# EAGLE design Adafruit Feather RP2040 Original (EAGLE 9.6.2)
COMPANY: ADAFRUIT INDUSTRIES; DRAWN: KTOWN; REV: B
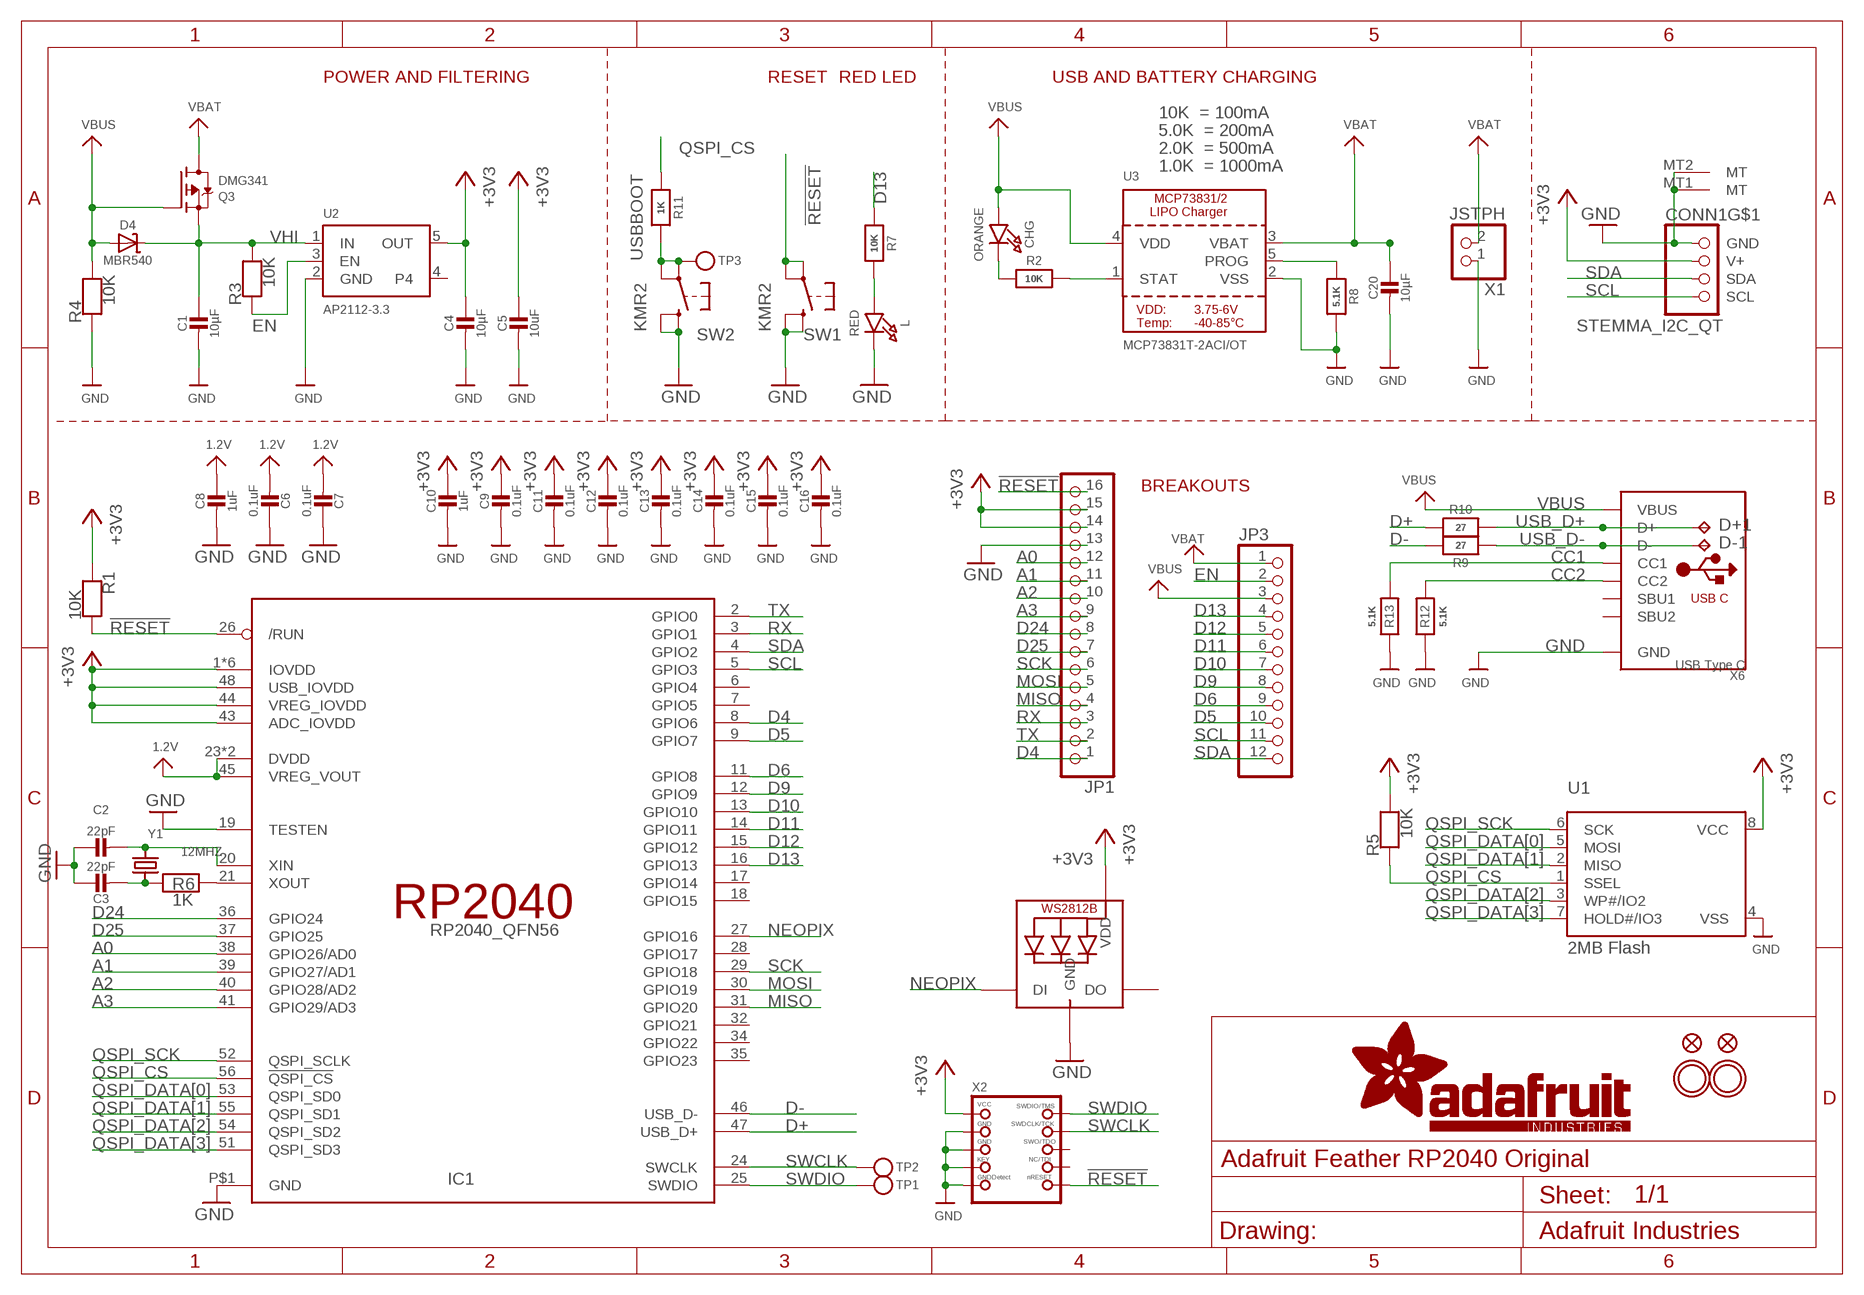
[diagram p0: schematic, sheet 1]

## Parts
C1  10µF  CAP_CERAMIC0805-NOOUTLINE  [0805-NO]
C2  22pF  CAP_CERAMIC0603_NO  [0603-NO]
C3  22pF  CAP_CERAMIC0603_NO  [0603-NO]
C4  10µF  CAP_CERAMIC0805-NOOUTLINE  [0805-NO]
C5  10uF  CAP_CERAMIC0805-NOOUTLINE  [0805-NO]
C6  0.1uF  CAP_CERAMIC0603_NO  [0603-NO]
C7  0.1uF  CAP_CERAMIC0603_NO  [0603-NO]
C8  1uF  CAP_CERAMIC0603_NO  [0603-NO]
C9  0.1uF  CAP_CERAMIC0603_NO  [0603-NO]
C10  1uF  CAP_CERAMIC0603_NO  [0603-NO]
C11  0.1uF  CAP_CERAMIC0603_NO  [0603-NO]
C12  0.1uF  CAP_CERAMIC0603_NO  [0603-NO]
C13  0.1uF  CAP_CERAMIC0603_NO  [0603-NO]
C14  0.1uF  CAP_CERAMIC0603_NO  [0603-NO]
C15  0.1uF  CAP_CERAMIC0603_NO  [0603-NO]
C16  0.1uF  CAP_CERAMIC0603_NO  [0603-NO]
C20  10µF  CAP_CERAMIC0805-NOOUTLINE  [0805-NO]
CHG  ORANGE  LED0603_NOOUTLINE  [CHIPLED_0603_NOOUTLINE]
CONN1  STEMMA_I2C_QT  [JST_SH4]
D4  MBR540  DIODE-SCHOTTKYSOD-123  [SOD-123]
D+1  TPB1,27  [B1,27]
D-1  TPB1,27  [B1,27]
IC1  RP2040_QFN56  [QFN56_7MM_REDUCEDEPAD]
JP1  HEADER-1X16ROUND  [1X16_ROUND]
JP3  HEADER-1X12  [1X12_ROUND]
L  RED  LED0603_NOOUTLINE  [CHIPLED_0603_NOOUTLINE]
LED1  WS2812B3535  [LED3535]
Q3  DMG341  MOSFET-P  [SOT23-R]
R1  10K  RESISTOR_0603_NOOUT  [0603-NO]
R2  10K  RESISTOR_0603_NOOUT  [0603-NO]
R3  10K  RESISTOR_0603_NOOUT  [0603-NO]
R4  10K  RESISTOR_0603_NOOUT  [0603-NO]
R5  10K  RESISTOR_0603_NOOUT  [0603-NO]
R6  1K  RESISTOR_0603_NOOUT  [0603-NO]
R7  10K  RESISTOR_0603_NOOUT  [0603-NO]
R8  5.1K  RESISTOR_0603_NOOUT  [0603-NO]
R9  27  RESISTOR_0603_NOOUT  [0603-NO]
R10  27  RESISTOR_0603_NOOUT  [0603-NO]
R11  1K  RESISTOR_0603_NOOUT  [0603-NO]
R12  5.1K  RESISTOR_0603_NOOUT  [0603-NO]
R13  5.1K  RESISTOR_0603_NOOUT  [0603-NO]
SW1  KMR2  SWITCH_TACT_SMT4.6X2.8  [BTN_KMR2_4.6X2.8]
SW2  KMR2  SWITCH_TACT_SMT4.6X2.8  [BTN_KMR2_4.6X2.8]
TP1  TESTPOINTROUND1.5MMNO  [TESTPOINT_ROUND_1.5MM_NO]
TP2  TESTPOINTROUND1.5MMNO  [TESTPOINT_ROUND_1.5MM_NO]
TP3  TESTPOINTROUND1.5MMNO  [TESTPOINT_ROUND_1.5MM_NO]
U1  2MB Flash  SPIFLASH_8PIN208MIL  [SOIC8_208MIL]
U2  AP2112-3.3  VREG_SOT23-5  [SOT23-5@1]
U3  MCP73831T-2ACI/OT  MCP73831/2  [SOT23-5]
U$31  MOUNTINGHOLE2.5  [MOUNTINGHOLE_2.5_PLATED]
U$32  MOUNTINGHOLE2.5  [MOUNTINGHOLE_2.5_PLATED]
U$34  FIDUCIAL_1MM  [FIDUCIAL_1MM]
U$35  FIDUCIAL_1MM  [FIDUCIAL_1MM]
X1  JSTPH  CON_JST_PH_2PIN_BATT  [JSTPH2_BATT]
X2  JTAG-CORTEXBOXPOSTS  [2X05_1.27MM_BOX_POSTS]
X6  USB Type C  USB_C  [USB_C_CUSB31-CFM2AX-01-X]
Y1  12MHZ  CRYSTAL2.5X2.0  [CRYSTAL_2.5X2]

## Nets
1.2V: C6.2 C7.2 C8.1 IC1.23(DVDD) IC1.45(VREG_VOUT) IC1.50(DVDD)
!RESET: IC1.26(/RUN) JP1.16 R1.2 SW1.A'(P1) SW1.A(P) X2.10(NRESET)
+3V3: C4.1 C5.1 C9.1 C10.1 C11.1 C12.1 C13.1 C14.1 C15.1 C16.1 CONN1.2(V+) IC1.1(IOVDD) IC1.10(IOVDD) IC1.22(IOVDD) IC1.33(IOVDD) IC1.42(IOVDD) IC1.43(ADC_IOVDD) IC1.44(VREG_IOVDD) IC1.48(USB_IOVDD) IC1.49(IOVDD) JP1.14 JP1.15 LED1.2(VDD) R1.1 R5.2 U1.8(VCC) U2.5(OUT) X2.1(VCC)
A0: IC1.38(GPIO26/AD0) JP1.12
A1: IC1.39(GPIO27/AD1) JP1.11
A2: IC1.40(GPIO28/AD2) JP1.10
A3: IC1.41(GPIO29/AD3) JP1.9
CC1: R13.2 X6.A5(CC1)
CC2: R12.2 X6.B5(CC2)
D4: IC1.8(GPIO6) JP1.1
D5: IC1.9(GPIO7) JP3.10
D6: IC1.11(GPIO8) JP3.9
D9: IC1.12(GPIO9) JP3.8
D10: IC1.13(GPIO10) JP3.7
D11: IC1.14(GPIO11) JP3.6
D12: IC1.15(GPIO12) JP3.5
D13: IC1.16(GPIO13) JP3.4 R7.1
D24: IC1.36(GPIO24) JP1.8
D25: IC1.37(GPIO25) JP1.7
D+: IC1.47(USB_D+) R10.2
D-: IC1.46(USB_D-) R9.2
EN: JP3.2 R3.1 U2.3(EN)
GND [power]: C1.2 C2.1 C3.1 C4.2 C5.2 C6.1 C7.1 C8.2 C9.2 C10.2 C11.2 C12.2 C13.2 C14.2 C15.2 C16.2 C20.2 CONN1.1(GND) CONN1.MT1(MT) CONN1.MT2(MT) IC1.19(TESTEN) IC1.P$1(GND) JP1.13 L.C LED1.4(GND) R4.1 R8.2 R12.1 R13.1 SW1.B'(S1) SW1.B(S) SW2.B'(S1) SW2.B(S) U1.4(VSS) U2.2(GND) U3.2(VSS) X1.1 X2.3(GND) X2.5(GND) X2.7(KEY) X2.9(GNDDETECT) X6.A1B12(GND) X6.B1A12(GND)
MISO: IC1.31(GPIO20) JP1.4
MOSI: IC1.30(GPIO19) JP1.5
N$1: CHG.C R2.1
N$2: L.A R7.2
N$3: R2.2 U3.1(STAT)
N$4: R8.1 U3.5(PROG)
N$5: C2.2 IC1.20(XIN) Y1.3
N$6: C3.2 R6.1 Y1.1
N$7: IC1.21(XOUT) R6.2
NEOPIX: IC1.27(GPIO16) LED1.1(DI)
QSPI_CS: IC1.56(!QSPI_CS) R5.1 R11.1 U1.1(SSEL)
QSPI_DATA[0]: IC1.53(QSPI_SD0) U1.5(MOSI)
QSPI_DATA[1]: IC1.55(QSPI_SD1) U1.2(MISO)
QSPI_DATA[2]: IC1.54(QSPI_SD2) U1.3(WP#/IO2)
QSPI_DATA[3]: IC1.51(QSPI_SD3) U1.7(HOLD#/IO3)
QSPI_SCK: IC1.52(QSPI_SCLK) U1.6(SCK)
RX: IC1.3(GPIO1) JP1.3
SCK: IC1.29(GPIO18) JP1.6
SCL: CONN1.4(SCL) IC1.5(GPIO3) JP3.11
SDA: CONN1.3(SDA) IC1.4(GPIO2) JP3.12
SWCLK: IC1.24(SWCLK) TP2.P$1 X2.4(SWDCLK)
SWDIO: IC1.25(SWDIO) TP1.P$1 X2.2(SWDIO)
TX: IC1.2(GPIO0) JP1.2
USB_D+: D+1.TP R10.1 X6.A6(D+) X6.B6(D+)
USB_D-: D-1.TP R9.1 X6.A7(D-) X6.B7(D-)
USBBOOT: R11.2 SW2.A'(P1) SW2.A(P) TP3.P$1
VBAT [power]: C20.1 JP3.1 Q3.3(D) U3.3(VBAT) X1.2
VBUS [power]: CHG.A D4.A JP3.3 Q3.1(G) R4.2 U3.4(VDD) X6.A4B9(VBUS) X6.B4A9(VBUS)
VHI [power]: C1.1 D4.C Q3.2(S) R3.2 U2.1(IN)
Unconnected: IC1.6(GPIO4) IC1.7(GPIO5) IC1.17(GPIO14) IC1.18(GPIO15) IC1.28(GPIO17) IC1.32(GPIO21) IC1.34(GPIO22) IC1.35(GPIO23) LED1.3(DO) U2.4 X2.6(SWO) X2.8(TDI) X6.A8(SBU1) X6.B8(SBU2)

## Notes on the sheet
- POWER AND FILTERING | RESET | RED LED | USB AND BATTERY CHARGING
- 10K  = 100mA
- 5.0K  = 200mA
- 2.0K  = 500mA
- 1.0K  = 1000mA
- BREAKOUTS

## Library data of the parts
C1-C3 C5-C16 C20 = microbuilder:CAP_CERAMIC: Ceramic Capacitors
C4 = microbuilder:CAP_CERAMIC: Ceramic Capacitors; REV: C
CHG L = microbuilder:LED: LED
CONN1 = microbuilder:STEMMA_I2C
D4 = microbuilder:DIODE-SCHOTTKY
D+1 D-1 = testpad:TP: Test pad
IC1 = adafruit_micro:RP2040
JP1 = microbuilder:HEADER-1X16: PIN HEADER
JP3 = microbuilder:HEADER-1X12
LED1 = microbuilder:WS2812B
Q3 = microbuilder:MOSFET-P: P-Channel Mosfet LEGEND VDS: Voltage Drain-Source ID: Drain Current RDS(ON): Drain-Source On-State Resistance VGS(TH): Gate-Source Threshold Voltage CISS: Drain-Source Input Capacitance SOT-23 Name VDS ID RDS(ON) VGS(TH) CISS Order Number IRLML5103 30V 760mA 600 mOhm -- 75pF @ 25V Digikey: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
R1-R13 = microbuilder:RESISTOR: Resistors
SW1 SW2 = microbuilder:SWITCH_TACT_SMT: SMT Tact Switches 6x6mm - Digikey: P12940SCT-ND KMR2 (4.6x2.8mm) - Digikey: 401-1426-1-ND EVQ-PQHB55 - Light Touch, 160GF (4.5x4.5mm) - Digikey: P8090SCT-ND KMT0 - KMT021 NGJ LHS (etc.) IP68/Waterproof - Digikey: CKN10289CT-ND
TP1-TP3 = microbuilder:TESTPOINT: Test Point
U1 = microbuilder:SPIFLASH_8PIN: SOIC8 SPI Flash Be careful with the size since SOIC8 flash comes in several 'widths' SOIC8 150 mil M25P16 - 16Mbit (2Mbit x 8) Serial Flash (75MHz SPI Bus), Supply: 2.7-3.6V Digikey: SOIC8 - M25P16-VMN6P-ND SOIC8 208 mil W25Q16BVSSIG - 16Mbit (2Mbit x 8) Serial Flash (104MHz SPI Bus), Supply: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
U2 = microbuilder:VREG_SOT23-5: SOT23-5 Fixed Voltage Regulators Part Current Out V Out V In V Dropout θJA (°C/W) TJ (°C) Digikey Part No. ADP121 150mA 3.3V 3.4-5.5V 0.09V @ 150mA -- -- ADP121-AUJZ33R7CT-ND ADP121 150mA 3.0V 3.1-5.5V 0.09V @ 150mA -- -- ADP121-AUJZ30R7CT-ND ADP122 300mA 3.3V 3.4-5.5V 0.085V @ 300mA -- --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
U3 = microbuilder:MCP73831/2: MCP73831/2 LIPO Charger VDD: 3.75 - 6V Temp -40 - 85°C Programmable Charge Rate: 15-500mA NOTE: STAT is a tri-state logic output on the MCP73831 and an open-drain output on the MCP73832. SOT23-5 with 4.2V output and tri-state logic on STAT = MCP73831T-2ACI/OT
U$31 U$32 = microbuilder:MOUNTINGHOLE: Mounting Hole; BOM: EXCLUDE
U$34 U$35 = microbuilder:FIDUCIAL: Fiducial Alignment Points; BOM: EXCLUDE
X1 = microbuilder:CON_JST_PH_2PIN: JST 2-Pin Right-Angle Connector
X2 = microbuilder:JTAG-CORTEX: Serial Wire (SW-DP) Connector Standard 0.05" 10-pin connector is for use with the Cortex M and Cortex A SWD (serial wire debugger) interface (SW-DP) Connectors 2x05_1.27MM_SMT - Inexpensive surface-mount header with bare pins, compatible with standard 10-pin SWD cables (4UCON: 16846)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
X6 = microbuilder:USB_C: USB Type-C USB 2.0 Connector
Y1 = microbuilder:CRYSTAL: Crystals

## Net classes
1 power: width 0.305 mm
2 gnd: width 0.254 mm

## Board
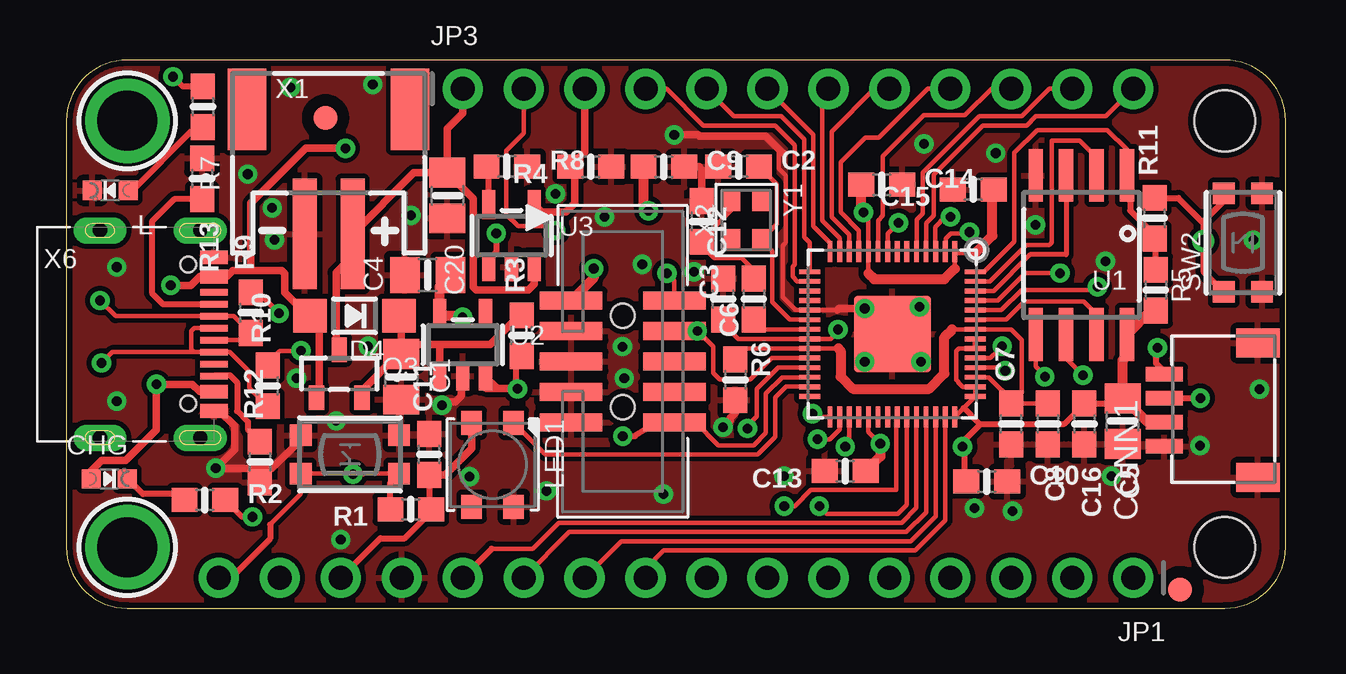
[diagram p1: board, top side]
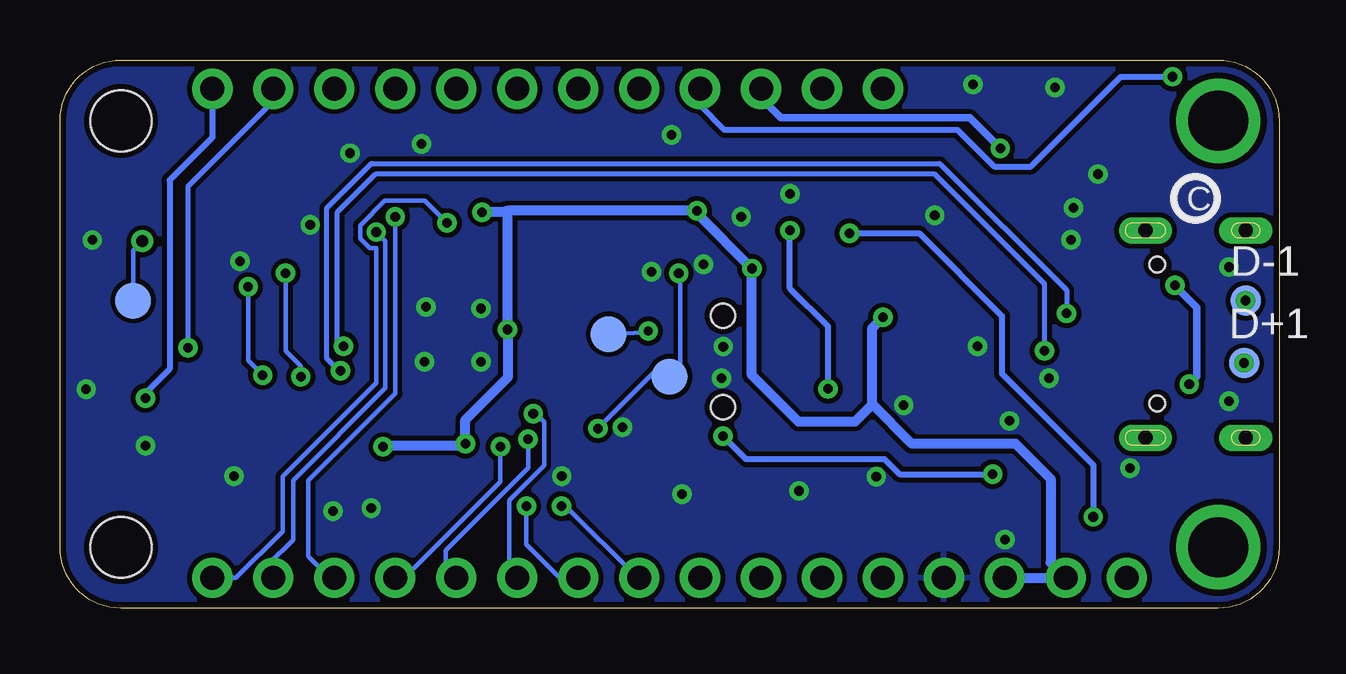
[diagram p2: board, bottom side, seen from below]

Size 50.8 x 22.86 mm. Coordinates in mm from the lower left corner, seen from the top.
Outline: 2.54,0 48.26,0 arc90 50.8,2.54 50.8,20.32 arc90 48.26,22.86 2.54,22.86 arc90 0,20.32 0,2.54 arc90 2.54,0
Copper layers (1*16): Top 0.035mm / dielectric 1.5mm / Bottom 0.035mm
Design rules "adafruit 7-7 *": minimum track width 7mil, minimum drill 15.5mil, track to track 8mil, track to pad 7mil, pad to pad 7mil, via to via 7mil, smd to smd 7mil, copper to edge 10mil, drill to drill 8mil, minimum pad ring 10mil, minimum via ring 8mil, stop-mask expansion 2mil, vias tented up to drill 20mil, thermal gap 10mil
Holes 2.54 mm at 48.26,20.32 48.26,2.54

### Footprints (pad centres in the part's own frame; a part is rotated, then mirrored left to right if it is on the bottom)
0805-NO = smd 1.24 x 1.5: 1 -0.95,0; 2 0.95,0
0603-NO = smd 1.075 x 1: 1 -0.85,0; 2 0.85,0
CHIPLED_0603_NOOUTLINE = smd 0.8 x 0.8: A 0,-0.75; C 0,0.75
JST_SH4 = smd 0.6 x 1.55: 1 -1.5,2.514; 2 -0.5,2.514; 3 0.5,2.514; 4 1.5,2.514 | smd 1.2 x 1.8: MT1 -2.8,-1.386; MT2 2.8,-1.386
SOD-123 = smd 1.4 x 1.4: A 1.85,0; C -1.85,0
B1,27 = smd 1.27 x 1.27: TP 0,0
QFN56_7MM_REDUCEDEPAD = smd 0.875 x 0.2: 1 -3.45,2.6; 2 -3.45,2.2; 3 -3.45,1.8; 4 -3.45,1.4; 5 -3.45,1; 6 -3.45,0.6; 7 -3.45,0.2; 8 -3.45,-0.2; 9 -3.45,-0.6; 10 -3.45,-1; 11 -3.45,-1.4; 12 -3.45,-1.8; 13 -3.45,-2.2; 14 -3.45,-2.6; 29 3.45,-2.6; 30 3.45,-2.2; 31 3.45,-1.8; 32 3.45,-1.4; 33 3.45,-1; 34 3.45,-0.6; 35 3.45,-0.2; 36 3.45,0.2; 37 3.45,0.6; 38 3.45,1; 39 3.45,1.4; 40 3.45,1.8; 41 3.45,2.2; 42 3.45,2.6 | smd 0.2 x 0.875: 15 -2.6,-3.45; 16 -2.2,-3.45; 17 -1.8,-3.45; 18 -1.4,-3.45; 19 -1,-3.45; 20 -0.6,-3.45; 21 -0.2,-3.45; 22 0.2,-3.45; 23 0.6,-3.45; 24 1,-3.45; 25 1.4,-3.45; 26 1.8,-3.45; 27 2.2,-3.45; 28 2.6,-3.45; 43 2.6,3.45; 44 2.2,3.45; 45 1.8,3.45; 46 1.4,3.45; 47 1,3.45; 48 0.6,3.45; 49 0.2,3.45; 50 -0.2,3.45; 51 -0.6,3.45; 52 -1,3.45; 53 -1.4,3.45; 54 -1.8,3.45; 55 -2.2,3.45; 56 -2.6,3.45 | smd 3.2 x 3.2: P$1 0,0
1X16_ROUND = drill 1 pad 1.676: 1 -19.05,0; 2 -16.51,0; 3 -13.97,0; 4 -11.43,0; 5 -8.89,0; 6 -6.35,0; 7 -3.81,0; 8 -1.27,0; 9 1.27,0; 10 3.81,0; 11 6.35,0; 12 8.89,0; 13 11.43,0; 14 13.97,0; 15 16.51,0; 16 19.05,0
1X12_ROUND = drill 1 pad 1.676: 1 -13.97,0; 2 -11.43,0; 3 -8.89,0; 4 -6.35,0; 5 -3.81,0; 6 -1.27,0; 7 1.27,0; 8 3.81,0; 9 6.35,0; 10 8.89,0; 11 11.43,0; 12 13.97,0
LED3535 = smd 1 x 0.85: 1 -1.75,0.875; 2 -1.75,-0.875; 3 1.75,-0.875; 4 1.75,0.875
SOT23-R = smd 0.635 x 1.016: 1 -0.95,-1; 2 0.95,-1; 3 0,1
BTN_KMR2_4.6X2.8 = smd 0.9 x 0.9: A 2.05,0.8; A' -2.05,0.8; B 2.05,-0.8; B' -2.05,-0.8
TESTPOINT_ROUND_1.5MM_NO = smd 1.5 x 1.5: P$1 0,0
SOIC8_208MIL = smd 0.6 x 2.2: 1 -1.905,-3.315; 2 -0.635,-3.315; 3 0.635,-3.315; 4 1.905,-3.315; 5 1.905,3.315; 6 0.635,3.315; 7 -0.635,3.315; 8 -1.905,3.315
SOT23-5@1 = smd 0.55 x 1.2: 1 -0.95,-1.3; 2 0,-1.3; 3 0.95,-1.3; 4 0.95,1.3; 5 -0.95,1.3
SOT23-5 = smd 0.55 x 1.2: 1 -0.95,-1.3; 2 0,-1.3; 3 0.95,-1.3; 4 0.95,1.3; 5 -0.95,1.3
MOUNTINGHOLE_2.5_PLATED = drill 2.5 pad 3.2: P$1 0,0
FIDUCIAL_1MM = smd 1 x 1: 1 0,0
JSTPH2_BATT = smd 1 x 4.6: 1 -1,-3.7; 2 1,-3.7 | smd 1.6 x 3.4: NC1 -3.4,1.5; NC2 3.4,1.5
2X05_1.27MM_BOX_POSTS = smd 0.76 x 2.6: 1 -2.54,-2.15; 2 -2.54,2.15; 3 -1.27,-2.15; 4 -1.27,2.15; 5 0,-2.15; 6 0,2.15; 7 1.27,-2.15; 8 1.27,2.15; 9 2.54,-2.15; 10 2.54,2.15 | hole 1: -1.905,0; 1.905,0
USB_C_CUSB31-CFM2AX-01-X = smd 0.575 x 1.15: A1B12 -3.2,3.545; A4B9 -2.4,3.545; B1A12 3.2,3.545; B4A9 2.4,3.545 | smd 0.275 x 1.15: A5 -1.25,3.545; A6 -0.25,3.545; A7 0.25,3.545; A8 1.25,3.545; B5 1.75,3.545; B6 0.75,3.545; B7 -0.75,3.545; B8 -1.75,3.545 | drill 0.6 pad 1 long: M1 -4.32,2.97; M2 4.32,2.97; M3 -4.32,-1.21; M4 4.32,-1.21 | hole 0.65: 2.89,2.47; -2.89,2.47
CRYSTAL_2.5X2 = smd 0.9 x 0.75: 1 -0.825,-0.625; 2 0.825,-0.625; 3 0.825,0.625; 4 -0.825,0.625

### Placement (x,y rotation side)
C1  13.95,9.65 270 top
C2  28,18.41 0 top
C3  26.48,16.13 270 top
C4  15.05,13.89 180 top
C5  44.01,7.8 270 top
C6  27.88,9.53 90 top
C7  39.37,7.68 90 top
C8  40.89,7.68 270 top
C9  24.89,18.4 0 top
C10  38.35,5.28 0 top
C11  15.11,6.41 90 top
C12  27.37,12.89 90 top
C13  32.45,5.71 180 top
C14  33.97,17.65 0 top
C15  37.78,17.46 180 top
C16  42.42,7.68 270 top
C20  15.88,17.21 270 top
CHG  1.78,5.4 270 top
CONN1  48.26,8.26 90 top
D4  12,12.19 180 top
D+1  1.46,10.22 0 bottom
D-1  1.4,12.83 0 bottom
IC1  34.42,11.43 270 top
JP1  25.4,1.27 180 top
JP3  30.48,21.65 0 top
L  1.82,17.42 90 top
LED1  17.75,5.98 270 top
Q3  11.37,9.78 0 top
R1  14.35,4.13 180 top
R2  5.77,4.51 0 top
R3  18.96,11.37 90 top
R4  21.84,18.41 180 top
R5  45.39,13.26 270 top
R6  28.64,12.89 270 top
R7  5.69,20.9 270 top
R8  18.35,18.41 0 top
R9  7.68,12.32 90 top
R10  8.38,9.27 90 top
R11  45.34,16.26 90 top
R12  8.06,6.1 90 top
R13  5.65,17.91 270 top
SW1  11.81,6.41 180 top
SW2  49.02,15.24 90 top
TP1  25.4,9.65 0 bottom
TP2  27.94,11.43 0 bottom
TP3  47.75,12.83 0 bottom
U1  42.29,14.73 180 top
U2  16.51,10.99 0 top
U3  18.54,15.53 0 top
U$1  [RP2040_BOT]  50.8,0 0 bottom
U$13  [PCBFEAT-REV-040]  3.49,17.08 0 bottom
U$31  2.54,20.32 270 top
U$32  2.54,2.54 270 top
U$34  10.79,20.45 270 top
U$35  46.4,0.77 270 top
U$43  [RP2040_TOP]  0,0 0 top
X1  10.92,19.3 0 top
X2  23.18,10.29 270 top
X6  2.6,11.43 270 top
Y1  28.32,16.19 270 top

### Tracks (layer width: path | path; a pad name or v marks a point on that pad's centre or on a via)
1.2V
  Top 0.178: 36.9,11.63 IC1.50 39.36,11.63 39.81,11.18 39.81,8.98 39.45,8.62 | 32.16,10.83 IC1.23 28.33,10.83 C6.2 | 39.45,8.62 C7.2 C8.1 | IC1.45 38.44,9.63 39.45,8.62
  Top 0.406: 36.9,11.63 36.58,11.3 36.58,9.78 35.94,9.14 32.77,9.14 32.26,9.65 32.26,10.73 32.16,10.83
!RESET  (via drill 0.4)
  Top 0.178: 12.38,5.61 SW1.A 9.76,4.77 8.48,3.49 | 12.38,5.61 SW1.A' | v11.94,5.59 12.36,5.59 12.38,5.61 | X2.10 26.23,7.75 26.69,7.29 26.69,7.27 27.16,6.79 28.64,6.79 29.15,7.3 29.15,8.95 29.82,9.63 IC1.26
  Top 0.254: JP1.16 6.86,1.27 8.48,2.9 8.48,3.49 | v23.18,7.18 23.68,7.18 24.64,7.77 24.69,7.75 X2.10 | R1.2 13.5,5.25 SW1.A'
  Bottom 0.254: v11.94,5.59 15.81,5.59 16.45,6.22 22.23,6.22 v23.18,7.18
+3V3  (via drill 0.4)
  Top 0.178: IC1.42 37.38,8.34 IC1.43 IC1.44 37.35,9.23 37.16,9.42 37.16,9.45 37.08,9.53 37.08,10.73 37.18,10.83 IC1.48 | IC1.33 33.42,7.35 v33.91,6.86 | 33.42,13.95 IC1.10 33.42,16.51 v33.21,16.51 | 37.02,14.16 IC1.1 37.08,14.82 37.87,14.82 | v32.15,11.62 32.15,11.53 31.86,11.23 IC1.22 27.99,11.23 27.37,11.85 C12.1 | C15.1 38.57,17.46 38.39,17.29
  Top 0.203: IC1.48 IC1.49
  Top 0.254: JP1.14 13.08,2.92 14.1,2.92 15.2,4.03 R1.1 15.11,4.21 C11.1 | 38.03,7.69 38.07,7.65 37.47,7.05 37.47,6.86 v37.34,6.73 37.4,6.67 37.4,5.5 C10.1 | 38.03,7.69 37.38,8.34 | 38.03,7.69 41.58,7.69 C16.1 43.79,8.53 C5.1
  Top 0.305: U2.5 15.65,12.19 | 16.45,12.19 v16.51,12.13 | 15.56,13.45 C4.1 | 24.04,16.79 v24.26,16.57 | LED1.2 16.88,6.66 15.79,5.56 C11.1
  Top 0.406: 16.45,12.19 15.65,12.19 | 33.42,13.95 33.66,13.72 36.58,13.72 37.02,14.16 | v33.21,16.51 33.12,16.6 C14.1 | v21.97,14.16 21.97,13.77 X2.1 | 37.87,14.82 38.58,15.53 38.58,17.1 38.39,17.29 | v33.91,6.86 33.91,6.33 C13.1 | CONN1.2 45.06,7.75 44.07,8.75 C5.1 44.01,10.34 44.26,10.59 44.26,11.35 U1.8 45.19,12.41 R5.2 | U2.5 15.56,13.45 | C9.1 24.04,16.79
  Bottom 0.178: 33.91,6.79 v33.91,6.86 | 32.15,16.57 32.19,16.57
  Bottom 0.305: 16.95,8.49 16.95,8.51
  Bottom 0.406: v16.51,12.13 16.95,11.68 16.95,8.51 15.3,6.86 10.99,6.86 9.53,5.4 9.53,1.91 JP1.15 JP1.14 | v37.34,6.73 37.27,6.79 33.91,6.79 | 32.19,16.57 32.26,16.51 v33.21,16.51 | v33.91,6.86 33.91,7.86 32.15,9.61 v32.15,11.62 32.15,16.57 v24.26,16.57 24.26,16.45 v21.97,14.16 21.97,9.72 20.03,7.78 17.67,7.78 16.95,8.49
A0
  Top 0.178: IC1.38 35.42,4.17 34.8,3.56 20.51,3.56 19.43,2.48 17.72,2.48
  Top 0.254: 17.72,2.48 JP1.12
A1
  Top 0.178: JP1.11 20.95,3.17 34.99,3.17 35.82,4 IC1.39
A2
  Top 0.178: IC1.40 36.22,3.83 35.18,2.79 23.11,2.79 JP1.10
A3
  Top 0.178: IC1.41 36.62,3.66 35.37,2.41 24.89,2.41 24.13,1.65 JP1.9
CC1
  Top 0.254: R13.2 4.48,17.06 3.56,16.13 3.56,13.14 4.02,12.68 X6.A5
CC2
  Top 0.254: X6.B5 6.18,9.71 6.82,9.71 7.11,9.42 7.11,8.22 7.56,7.77 7.56,7.45 R12.2
D4  (via drill 0.39)
  Top 0.178: IC1.8 34.22,15.61 v34.67,16.07
  Bottom 0.178: v34.67,16.07 35.59,16.99 37.26,16.99 38.29,15.96 38.29,15.41 37.9,15.02 37.62,15.02 37.62,9.4 41.53,5.49 41.53,3.21 43.47,1.27 JP1.1
D5
  Top 0.178: JP3.10 38.54,21.65 37.44,20.55 35.73,20.55 34.02,18.84 34.02,16.37 33.82,16.17 IC1.9
D6
  Top 0.178: JP3.9 35.88,21.65 33.85,19.62 33.27,19.62 32.26,18.61 32.26,16.51 33.02,15.75 IC1.11
D9
  Top 0.178: JP3.8 33.66,21.65 31.88,19.88 31.88,16.32 32.62,15.58 IC1.12
D10
  Top 0.178: IC1.13 32.22,15.44 31.5,16.16 31.5,21.4 JP3.7
D11
  Top 0.178: JP3.6 31.12,19.75 31.12,15.93 31.82,15.23 IC1.14
D12
  Top 0.178: JP3.5 27.81,20.51 29.79,20.51 30.74,19.56 30.74,15.47 30.97,15.24 IC1.15
D13  (via drill 0.4)
  Top 0.178: JP3.4 25.02,21.65 26.54,20.13 29.53,20.13 30.35,19.31 30.35,14.33 30.26,14.24 30.26,13.82 30.45,13.63 IC1.16
  Top 0.254: R7.1 4.85,21.75 v4.45,22.16
  Bottom 0.254: v4.45,22.16 6.6,22.16 10.35,18.41 11.87,18.41 13.4,19.94 23.11,19.94 24.13,20.95 JP3.4
D24  (via drill 0.4)
  Top 0.178: IC1.36 34.58,7.95 34.58,4.92 31.02,4.92 30.35,4.25 v29.91,4.25
  Bottom 0.178: v29.91,4.25 29.72,4.25 26.73,1.27 JP1.8
D25  (via drill 0.4)
  Top 0.178: IC1.37 35.02,4.31 34.64,3.94 31.69,3.94 v31.37,4.25
  Bottom 0.178: JP1.7 29.97,1.27 31.37,2.67 31.37,4 v31.37,4.25
D+  (via drill 0.4)
  Top 0.178: v9.78,10.73 8.89,10.73 8.38,10.22 R10.2 | IC1.47 38.5,10.43 38.8,10.73 v38.99,10.92
  Bottom 0.203: v38.99,10.92 39.05,10.92 39.24,11.11 39.24,16.51 37.66,18.1 14.35,18.1 9.78,13.53 v9.78,10.73
D-  (via drill 0.4)
  Top 0.178: v39.12,9.91 38.99,10.03 IC1.46
  Top 0.203: v8.86,12.29 7.98,13.17 R9.2
  Bottom 0.203: v39.12,9.91 39.18,9.91 39.69,10.41 39.69,16.68 37.82,18.54 14.14,18.54 8.86,13.26 v8.86,12.29
EN  (via drill 0.4)
  Top 0.178: JP3.2 19.05,19.8 18.33,19.09 18.33,16.42 18.82,15.94 20.19,15.94 v20.38,15.75
  Top 0.254: R3.1 18.73,10.29 18.73,9.18 17.96,9.18 U2.3 17.46,9.14 v18.8,9.14
  Bottom 0.254: v18.8,9.14 18.8,11.75 20.38,13.34 v20.38,15.75
GND  (via drill 0.39, 0.4)
  Top 0.178: 32.11,12.43 IC1.19 30.39,12.43 29.84,12.98 29.84,15.11 29.97,15.24 29.97,18.03 29.69,18.32 29.69,19.14
  Top 0.305: U2.2 16.45,9.62 16.45,8.86 16.19,8.61 15.65,8.61 v15.65,8.47 | SW1.B 9.76,7.02 8.56,5.82 6.22,5.82 7.01,6.61 7.01,7.59 6.38,8.23 X6.B1A12 | 32.11,12.43 32.18,12.5 v33.26,12.5 34.33,11.43 IC1.P$1 | C6.1 27.88,8.15 27.65,7.92 27.65,7.84 v27.36,7.54 | C3.1 26.48,18.29 26.36,18.4 C9.2 | v25.32,19.74 26.31,19.74 26.36,19.68 29.15,19.68 29.69,19.14 29.91,18.92
  other vias: 11.24,7.81 23.24,9.59 14.35,16.38 8.57,16.7 6.22,5.84 9.33,21.72 12.76,21.84 12.57,10.92 7.56,18.1 16.79,5.49 8.67,15.35 26.15,14.02 23.99,14.34 23.16,10.91 24.88,4.75 35.55,12.56 35.61,10.27 33.26,10.27 35.74,19.35 43.29,14.47 37.83,4.18 49.71,9.13 47.23,6.78 43.55,5.51 22.42,16.32 20.38,17.27 38.72,18.97 9.59,9.59 2.1,8.64 2.1,14.22 20,4.89 11.43,2.86 49.45,15.35 39.42,4.05 29.9,5.51 40.37,15.99
  pour Top: 0,22.86 0,0 50.8,-0.06 50.8,22.86
  pour Bottom: 50.93,0 0,0 0,22.86 50.93,22.86
MISO  (via drill 0.4)
  Top 0.178: IC1.31 32.62,6.9 v32.45,6.73
  Bottom 0.178: v32.45,6.73 32.45,5.27 36.45,1.27 JP1.4
MOSI  (via drill 0.4)
  Top 0.178: IC1.30 32.22,7.46 31.81,7.05 v31.3,7.05
  Bottom 0.178: v31.3,7.05 31.3,5.85 34.73,2.41 34.73,1.52 34.48,1.27 JP1.5
N$1
  Top 0.254: R2.1 4.66,4.76 3.18,4.76 2.54,5.4 CHG.C
N$2
  Top 0.254: R7.2 5.52,19.89 5.2,19.89 2.74,17.42 L.A
N$3  (via drill 0.4)
  Top 0.254: v7.75,3.81 7.31,3.81 R2.2 | v17.91,15.63 17.91,14.84 17.59,14.53 U3.1
  Bottom 0.254: v7.75,3.81 7.75,5.97 11.56,9.78 11.56,12.19 15,15.63 v17.91,15.63
N$4
  Top 0.254: R8.1 17.57,18.35 17.57,16.86 U3.5
N$5
  Top 0.178: C2.2 29.59,17.68 29.59,16.01 Y1.3 29.41,14.9 29.41,12.76 30.14,12.03 IC1.20
N$6
  Top 0.178: Y1.1 27.7,16.59 26.48,15.37 C3.2 26.48,15.13 27,14.61 28.13,14.61 28.64,14.1 R6.1
N$7
  Top 0.178: IC1.21 29.05,11.63 R6.2
NEOPIX
  Top 0.178: LED1.1 19.95,6.41 28.8,6.41 29.53,7.14 29.53,8.79 29.98,9.25 30.95,9.25 IC1.27
QSPI_CS
  Top 0.178: IC1.56 38.25,14.03 39.5,15.28 39.5,18.99 40.45,19.94 43.37,19.94 44.2,19.11 U1.1 44.2,17.08 44.32,16.95
  Top 0.254: R5.1 45.39,15.14 45.58,15.33 | 45.58,15.33 45.64,15.39 45.35,15.39 R11.1 | 44.32,16.95 44.32,16.59 45.58,15.33
QSPI_DATA[0]  (via drill 0.39)
  Top 0.178: IC1.53 38.8,12.83 39.94,13.97 v41.4,13.97 | v40.77,9.65 40.77,9.7 40.39,10.08 U1.5
  Bottom 0.178: v41.4,13.97 41.4,10.73 40.77,10.1 v40.77,9.65
QSPI_DATA[1]
  Top 0.178: 42.93,18.8 42.23,19.49 41.05,19.49 41.05,15.24 40.96,15.14 39.98,15.14 38.47,13.63 IC1.55
  Top 0.203: 42.93,18.8 U1.2
QSPI_DATA[2]
  Top 0.178: IC1.54 38.63,13.23 40.15,14.74
  Top 0.203: U1.3 41.66,14.74 40.15,14.74
QSPI_DATA[3]
  Top 0.178: IC1.51 39.16,12.03 39.91,12.78 42.4,12.78 42.93,12.26 U1.7
QSPI_SCK  (via drill 0.39)
  Top 0.178: IC1.52 38.95,12.43 39.8,13.27 42.83,13.27 v42.96,13.4 | v42.35,9.72 41.66,10.41 U1.6
  Bottom 0.178: v42.96,13.4 42.96,10.32 v42.35,9.72
RX  (via drill 0.4)
  Top 0.178: v36.83,16.32 36.62,16.32 36.2,15.89 36.2,14.9 IC1.3
  Bottom 0.178: JP1.3 39.56,1.27 40.45,2.16 40.45,5.33 36.83,8.95 v36.83,16.32
SCK  (via drill 0.4)
  Top 0.178: IC1.29 31.21,7.98 v31.08,8.11
  Bottom 0.178: v31.08,8.11 30.98,8.11 30.63,7.76 30.63,5.95 32.09,4.49 32.09,1.42 31.94,1.27 JP1.6
SCL  (via drill 0.4)
  Top 0.178: JP3.11 40.96,21.65 39.81,20.51 38.03,20.51 35.68,18.17 35.68,16.46 35.44,16.21 35.44,14.9 IC1.5
  Top 0.254: CONN1.4 45.81,9.82 45.41,10.21 45.4,10.79 v45.47,10.86
  Bottom 0.203: v45.47,10.86 45.47,17.59 41.91,21.14 JP3.11
SDA  (via drill 0.4)
  Top 0.178: JP3.12 43.31,20.51 40.39,20.51 40.01,20.13 38.19,20.13 36.13,18.07 36.13,16.36 35.82,16.05 IC1.4
  Top 0.254: v47.24,8.76 47.02,8.76 CONN1.3
  Bottom 0.254: JP3.12 44.45,19.62 46.23,17.84 46.23,9.97 47.24,8.95 v47.24,8.76
SWCLK  (via drill 0.39)
  Top 0.178: IC1.24 29.38,10.43 28.49,9.54 27.22,9.54 26.96,9.8 26.96,10.9 26.3,11.56 v26.29,11.56 X2.4
  Bottom 0.178: TP2.P$1 26.35,11.49 v26.29,11.56
SWDIO  (via drill 0.4)
  Top 0.178: X2.2 25.33,13.66 v25.02,13.97 | v28.38,7.49 28.38,7.62 28.77,8 28.77,9.14 29.65,10.03 IC1.25
  Bottom 0.178: v25.02,13.97 24.96,13.91 24.96,10.1 TP1.P$1 25.59,9.84 25.59,9.91 25.97,9.91 v28.38,7.49
TX  (via drill 0.4)
  Top 0.178: IC1.2 36.64,14.9 36.64,15.41 36.84,15.62 37.56,15.62 v37.62,15.68
  Bottom 0.178: v37.62,15.68 37.24,15.3 37.24,9.18 41.08,5.33 41.08,2.86 42.1,1.84 42.1,1.4 41.97,1.27 JP1.2
USB_D+  (via drill 0.4)
  Top 0.178: 5.32,10.68 X6.B6 6.8,10.68 7.62,9.87 7.62,9.19 R10.1 | 5.32,10.68 5.21,10.79 5.21,11.56 5.33,11.68 X6.A6 | 5.32,10.68 1.92,10.68 D+1.TP
  other vias: 1.46,10.22
USB_D-  (via drill 0.4)
  Top 0.178: X6.A7 7.39,11.18 R9.1 6.97,12.18 X6.B7 2.04,12.18 D-1.TP
  other vias: 1.4,12.83
USBBOOT  (via drill 0.5)
  Top 0.178: 47.37,15.18 v47.37,15.3
  Top 0.254: SW2.A 48.22,16.98 47.37,16.13 47.37,16.07 | 47.37,16.07 47.37,15.18 47.37,14.04 SW2.A' | R11.2 46.33,17.11 47.37,16.07
  Bottom 0.178: TP3.P$1 47.75,14.92 v47.37,15.3
VBAT
  Top 0.305: Q3.3 11.24,10.91 11.24,13.99 11.92,14.67 X1.2 14.48,18.16 C20.1 | JP3.1 16.51,20.64 15.88,20 C20.1 | C20.1 16.95,17.08 16.95,15.5 16.95,13.4 17.08,13.27 19.24,13.27 19.49,13.52 U3.3
VBUS  (via drill 0.4)
  Top 0.305: Q3.1 10.54,8.91 10.54,11.7 10.15,12.09 D4.A 10.06,12.19 10.06,12.2 9.09,13.17 9.09,13.96 8.97,14.09 7.68,14.09 | v4.34,13.46 5.19,13.46 5.56,13.83 X6.A4B9 6.68,13.83 6.93,14.09 7.68,14.09 | X6.B4A9 5.56,9.03 5.25,9.34 v3.75,9.34 3.75,7.43 2.48,6.16 1.47,6.16 1.03,5.71 CHG.A | v11.62,19.18 9.97,19.18 7.68,16.89 7.68,14.09 | JP3.3 21.59,19.01 R4.2 21.18,18.22 21.18,16.89 20.81,16.52 19.81,16.52 U3.4
  Bottom 0.305: v4.34,13.46 3.43,12.55 3.43,9.65 v3.75,9.34 | JP3.3 21.59,21.27 20.77,20.45 12.89,20.45 v11.62,19.18
VHI
  Top 0.305: 15.56,10.99 17.65,10.99 18.88,12.22 R3.2 | U2.1 15.56,10.99 | C1.1 13.84,10.6 12.32,9.08 Q3.2 | C1.1 13.95,12.1 D4.C | 15.56,10.99 14.34,10.99 C1.1

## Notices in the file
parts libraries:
microbuilder: This work is placed in the public domain, and may be freely used for commercial and non-commercial work with the following conditions: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
